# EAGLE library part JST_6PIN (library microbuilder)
JST 6-Pin Right-Angle Connector
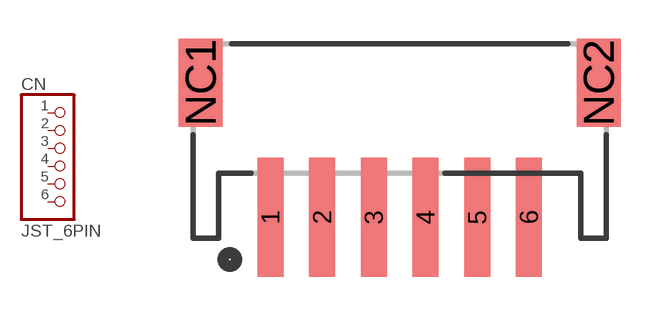
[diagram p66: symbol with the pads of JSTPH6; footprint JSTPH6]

Designator prefix CN

## JST_6PIN  [JSTPH6]
1  1  pas
2  2  pas
3  3  pas
4  4  pas
5  5  pas
6  6  pas

## Footprint JSTPH6 (pad centres in mm)
smd 1 x 4.6: 1 -5,-3.7; 2 -3,-3.7; 3 -1,-3.7; 4 1,-3.7; 5 3,-3.7; 6 5,-3.7
smd 1.7 x 3.4: NC1 -7.7,1.5; NC2 7.7,1.5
